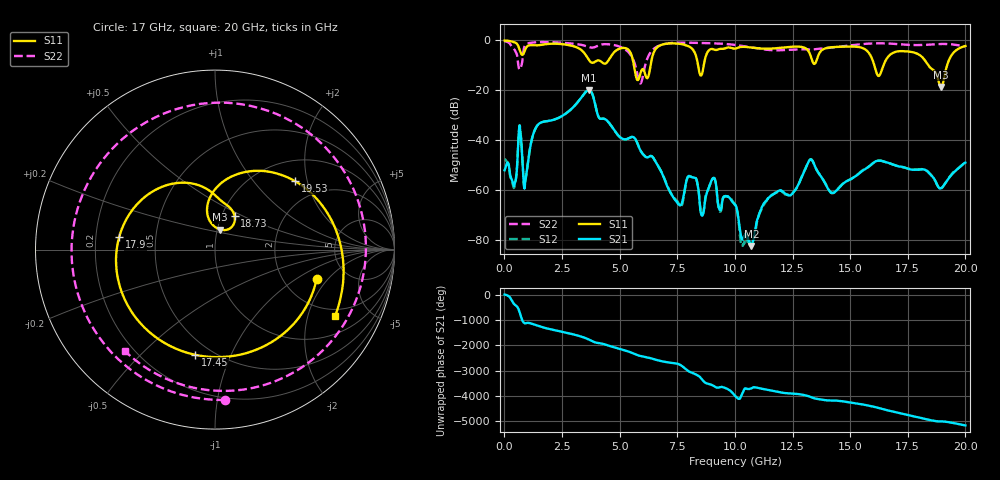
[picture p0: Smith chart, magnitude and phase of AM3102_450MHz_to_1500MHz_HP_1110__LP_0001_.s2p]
!Agilent Technologies,E8364B,MY43040894,A.07.50.67
!Agilent E8364B: A.07.50.67
!Date: Thursday, January 11, 2018 06:42:16
!Correction: S11(Full 2 Port(1,2))
!S21(Full 2 Port(1,2))
!S12(Full 2 Port(1,2))
!S22(Full 2 Port(1,2))
!S2P File: Measurements: S11, S21, S12, S22:
# Hz S  dB  R 50
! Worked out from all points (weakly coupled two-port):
!   1601 points, 10 MHz to 20 GHz, reference 50 ohm
!   highest |S21| = -20.02 dB at 3.671 GHz (marker M1); lowest = -82.6 dB at 10.72 GHz (marker M2)
!   lowest |S11| = -18.8 dB at 18.95 GHz (marker M3), VSWR 1.26, Z = 51.6 + j11.7 ohm
!   |S11| at or under -10 dB: 5.618 GHz to 6.345 GHz (726.5 MHz wide, 12.1 % of centre); 16.05 GHz to 16.45 GHz (401.3 MHz wide, 2.47 % of centre); 18.38 GHz to 19.21 GHz (823.1 MHz wide, 4.38 % of centre)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
!   |S22| runs from -17.4 to -0.3 dB; largest |S21 - S12| = 0.013
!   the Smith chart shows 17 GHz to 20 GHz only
!   S11 on the Smith chart (normalised r, x): 17 GHz: 3.03, -1.52; 17.45 GHz: 0.41, -0.74; 17.9 GHz: 0.30, +0.06; 18.73 GHz: 1.15, +0.45; 19.53 GHz: 1.46, +1.69; 20 GHz: 1.68, -3.00
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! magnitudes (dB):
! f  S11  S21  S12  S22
! 10 MHz  -0.1  -52.2  -47.7  -0.3
! 422.3 MHz  -0.8  -58.6  -59.1  -3.6
! 672.2 MHz  -4.2  -34.4  -34.3  -11.7
! 909.5 MHz  -3.7  -56.3  -56.6  -2.0
! 1.422 GHz  -2.1  -34.3  -34.3  -0.8
! 3.346 GHz  -4.0  -22.9  -22.9  -1.9
! 3.671 GHz  -8.0  -20.0  -20.0  -2.8
! 5.895 GHz  -13.5  -44.1  -44.1  -17.4
! 6.682 GHz  -2.5  -50.6  -50.6  -2.3
! 7.619 GHz  -1.5  -66.3  -66.4  -1.0
! 10.01 GHz  -3.4  -66.1  -66.1  -1.9
! 10.72 GHz  -3.0  -82.6  -82.2  -2.9
! 13.34 GHz  -7.8  -48.1  -48.0  -3.8
! 14.24 GHz  -2.8  -61.2  -61.4  -2.9
! 16.68 GHz  -6.4  -49.3  -49.3  -1.3
! 17 GHz  -4.6  -50.3  -50.3  -1.5
! 17.45 GHz  -4.5  -51.4  -51.3  -1.8
! 17.9 GHz  -5.4  -52.0  -51.9  -2.0
! 18.73 GHz  -13.3  -57.0  -57.1  -1.6
! 18.95 GHz  -18.8  -59.3  -59.5  -1.5
! 19.53 GHz  -4.6  -52.8  -52.6  -1.8
! 20 GHz  -2.3  -49.1  -49.3  -2.4
